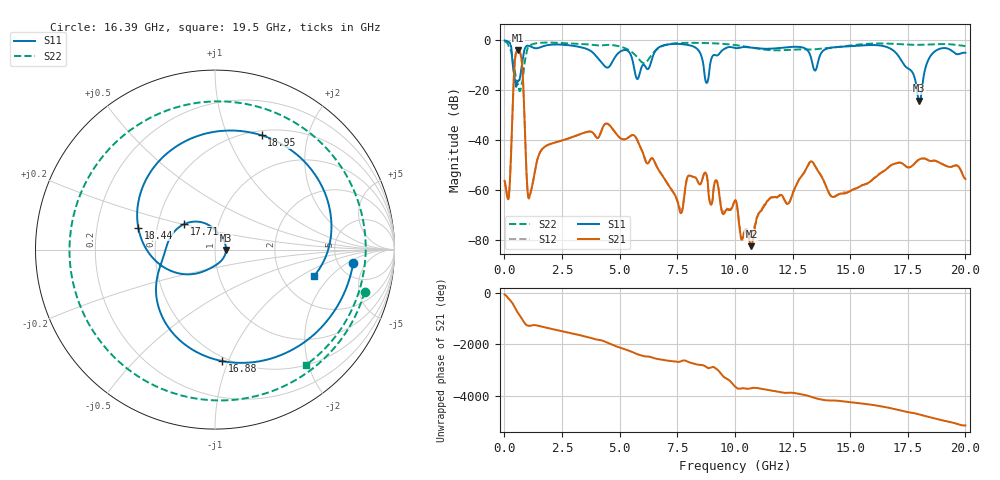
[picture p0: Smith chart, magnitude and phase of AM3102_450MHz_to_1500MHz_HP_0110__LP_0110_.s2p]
!Agilent Technologies,E8364B,MY43040894,A.07.50.67
!Agilent E8364B: A.07.50.67
!Date: Thursday, January 11, 2018 05:47:13
!Correction: S11(Full 2 Port(1,2))
!S21(Full 2 Port(1,2))
!S12(Full 2 Port(1,2))
!S22(Full 2 Port(1,2))
!S2P File: Measurements: S11, S21, S12, S22:
# Hz S  dB  R 50
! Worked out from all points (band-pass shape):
!   1601 points, 10 MHz to 20 GHz, reference 50 ohm
!   highest |S21| = -4.03 dB at 584.7 MHz (marker M1); lowest = -82.7 dB at 10.72 GHz (marker M2)
!   |S21| within 3 dB of the highest: 468.3 MHz to 734.2 MHz (265.9 MHz wide, 44.2 % of centre)
!   lowest |S11| = -24.2 dB at 18 GHz (marker M3), VSWR 1.13, Z = 56.5 - j0.17 ohm
!   |S11| at or under -10 dB: 364.7 MHz to 757.2 MHz (392.5 MHz wide, 70 % of centre); 5.605 GHz to 5.998 GHz (393 MHz wide, 6.77 % of centre); 17.35 GHz to 18.3 GHz (948.9 MHz wide, 5.32 % of centre)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
!   |S22| runs from -20.5 to -0.4 dB; largest |S21 - S12| = 0.0018
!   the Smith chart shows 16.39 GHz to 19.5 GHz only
!   S11 on the Smith chart (normalised r, x): 16.39 GHz: 6.89, -2.54; 16.88 GHz: 0.47, -0.95; 17.71 GHz: 0.68, +0.20; 18.44 GHz: 0.39, +0.12; 18.95 GHz: 0.55, +1.34; 19.5 GHz: 3.03, -1.32
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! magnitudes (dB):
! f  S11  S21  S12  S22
! 10 MHz  -0.1  -56.5  -56.3  -0.4
! 197.4 MHz  -0.7  -62.9  -61.9  -2.6
! 584.7 MHz  -16.2  -4.0  -4.0  -17.6
! 759.6 MHz  -9.9  -8.9  -8.9  -17.5
! 1.084 GHz  -2.3  -63.0  -63.2  -2.3
! 3.346 GHz  -2.9  -37.5  -37.5  -1.5
! 6.682 GHz  -3.0  -52.0  -52.0  -3.2
! 7.644 GHz  -1.5  -69.4  -68.1  -1.1
! 8.781 GHz  -17.1  -54.4  -54.4  -1.1
! 10.01 GHz  -3.1  -64.3  -64.5  -1.9
! 10.72 GHz  -3.0  -82.7  -78.5  -2.9
! 13.34 GHz  -8.4  -48.7  -48.7  -3.7
! 14.24 GHz  -2.9  -62.9  -63.0  -2.9
! 16.39 GHz  -2.2  -52.9  -52.9  -1.2
! 16.68 GHz  -3.0  -50.8  -50.9  -1.3
! 16.88 GHz  -4.1  -49.7  -49.7  -1.4
! 17.71 GHz  -13.1  -50.2  -50.3  -1.8
! 18 GHz  -24.2  -47.8  -47.8  -1.8
! 18.44 GHz  -7.0  -48.4  -48.4  -1.7
! 18.95 GHz  -3.2  -49.5  -49.5  -1.5
! 19.5 GHz  -4.9  -50.4  -50.4  -1.7
! 20 GHz  -5.0  -55.7  -55.5  -2.3
